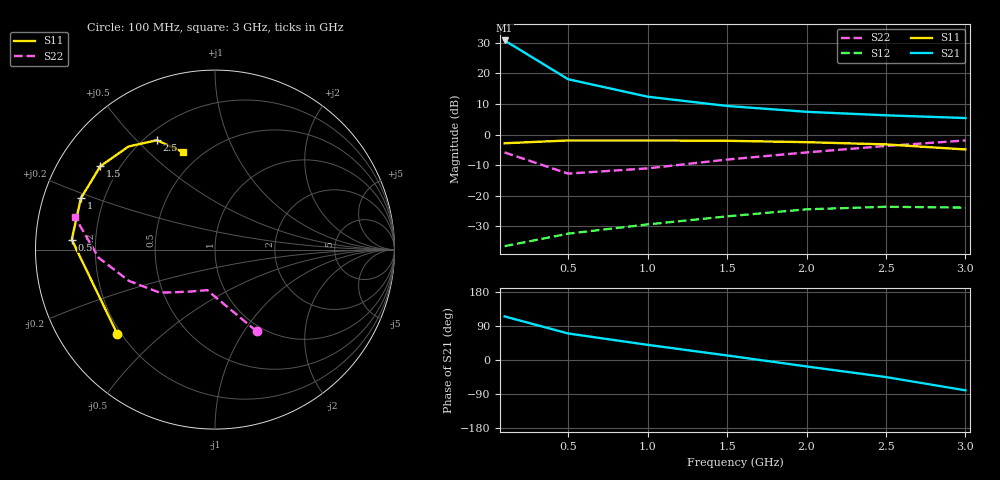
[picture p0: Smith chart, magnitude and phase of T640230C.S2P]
!AT-64023
!S-PARAMETERS at Vce=10V  Ic=110mA.  LAST UPDATED 06-28-94
# ghz s ma r 50
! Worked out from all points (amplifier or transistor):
!   7 points, 100 MHz to 3 GHz, reference 50 ohm
!   highest |S21| = 30.7 dB at 100 MHz (marker M1)
!   |S21| within 3 dB of that: start of sweep to 194.7 MHz
!   unconditionally stable (mu >= 1): 867.2 MHz to 1.636 GHz
!   at 500 MHz: K = 0.82, MSG = 25.2 dB, |S12| = -32.4 dB
!   at 1.5 GHz: K = 1.03, MAG = 17.0 dB, |S12| = -26.7 dB
!   at 3 GHz: K = 0.63, MSG = 14.6 dB, |S12| = -23.9 dB
!   S11 on the Smith chart (normalised r, x): 100 MHz: 0.18, -0.36; 500 MHz: 0.11, +0.03; 1 GHz: 0.11, +0.18; 1.5 GHz: 0.13, +0.32; 2.5 GHz: 0.25, +0.57; 3 GHz: 0.40, +0.65
0.1  0.72 -139.0  34.41 115.0  0.015 40.0  0.51 -63.0
0.5  0.8 176.0  8 70.0  0.024 34.0  0.23 -101.0
1  0.8 159.0  4.15 40.0  0.034 36.0  0.28 -123.0
1.5  0.79 144.0  2.93 12.0  0.046 34.0  0.39 -142.0
2  0.75 130.0  2.35 -17.0  0.06 21.0  0.51 -160.0
2.5  0.69 118.0  2.06 -45.0  0.066 10.0  0.65 -176.0
3  0.57 108.0  1.86 -80.0  0.064 -13.0  0.8 167.0
